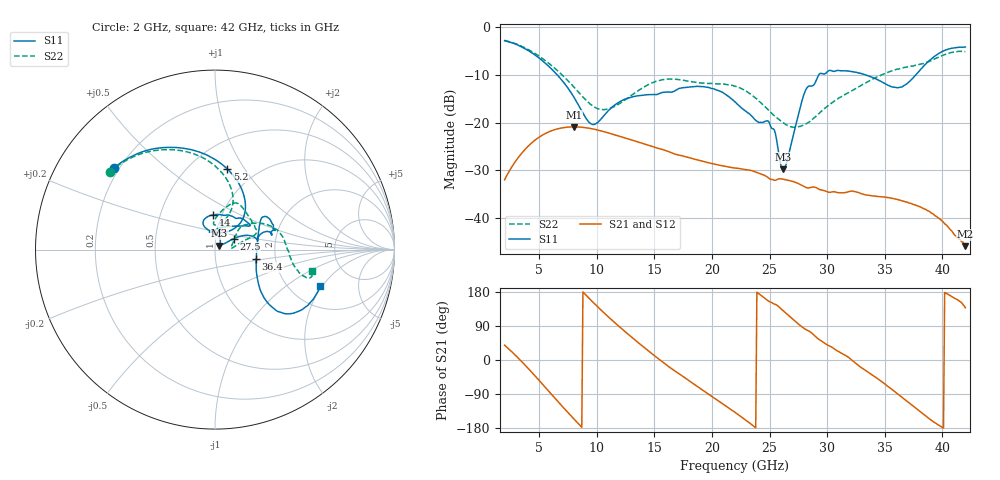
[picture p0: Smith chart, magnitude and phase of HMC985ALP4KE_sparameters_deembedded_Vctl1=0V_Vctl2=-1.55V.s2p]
!s2p File: Measurements: S11, S21, S12, S22
# GHz S dB R 50.0
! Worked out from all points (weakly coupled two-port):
!   401 points, 2 GHz to 42 GHz, reference 50 ohm
!   highest |S21| = -20.89 dB at 8 GHz (marker M1); lowest = -45.9 dB at 42 GHz (marker M2)
!   lowest |S11| = -29.8 dB at 26.2 GHz (marker M3), VSWR 1.07, Z = 52.4 + j2.31 ohm
!   |S11| at or under -10 dB: 6.574 GHz to 29.27 GHz (22.7 GHz wide, 127 % of centre); 33.36 GHz to 37.7 GHz (4.34 GHz wide, 12.2 % of centre)
!   |S22| runs from -21.0 to -2.8 dB; largest |S21 - S12| = 0.00016
!   S11 on the Smith chart (normalised r, x): 2 GHz: 0.18, +0.34; 5.2 GHz: 0.74, +0.84; 14 GHz: 0.91, +0.37; 27.5 GHz: 1.22, +0.15; 36.4 GHz: 1.58, -0.18; 42 GHz: 2.90, -1.91
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2  -2.80 141.0  -32.00 39.0  -32.00 39.0  -2.76 143.4
3.5  -4.14 113.4  -26.39 -4.7  -26.38 -4.7  -4.01 118.1
5.2  -6.85 81.3  -22.74 -60.8  -22.74 -60.8  -6.40 91.8
8  -14.59 46.3  -20.89 -155.1  -20.90 -155.1  -12.49 67.7
8.7  -17.59 52.0  -20.97 -177.5  -20.98 -177.5  -14.36 69.8
9.7  -20.40 84.2  -21.34 151.7  -21.35 151.7  -16.60 79.7
10.8  -18.04 112.0  -22.02 119.6  -22.02 119.6  -17.23 91.2
14  -14.24 92.5  -24.38 35.8  -24.38 35.8  -12.67 77.5
15.4  -13.94 73.0  -25.44 2.4  -25.45 2.4  -11.16 68.7
19.4  -12.52 34.4  -28.24 -83.8  -28.25 -83.8  -11.74 38.0
22  -15.64 52.3  -29.53 -138.0  -29.52 -138.1  -12.36 20.7
25  -20.14 98.1  -31.79 154.0  -31.80 154.0  -17.62 13.1
26.2  -29.78 42.9  -31.89 129.3  -31.89 129.3  -20.07 6.0
27.5  -18.37 29.9  -32.79 95.0  -32.81 95.0  -20.88 7.0
28.1  -13.34 20.8  -33.52 81.3  -33.53 81.5  -20.38 13.4
28.7  -12.30 12.9  -33.53 70.0  -33.52 70.0  -19.35 20.9
31  -9.07 23.3  -34.71 22.3  -34.73 22.0  -14.87 40.9
33.3  -9.95 34.3  -35.14 -26.6  -35.15 -26.7  -11.74 34.3
35.4  -12.27 12.3  -35.79 -72.5  -35.78 -72.6  -9.35 22.1
36.4  -12.57 -12.9  -36.34 -96.2  -36.34 -96.2  -8.58 15.0
39.5  -5.81 -43.3  -39.72 -167.9  -39.76 -168.2  -6.43 -14.2
42  -4.14 -19.0  -45.93 137.7  -45.84 137.4  -5.10 -12.3
